(* Logix 5000 AddOnInstructionDefinition export AMCI_3601_AOP_Home_CCW; software revision 20.03 *)

ADD_ON_INSTRUCTION AMCI_3601_AOP_Home_CCW   (* revision 0.0, vendor AMCI, ExecuteEnableInFalse *)
// Revision note:
// 3/2020: Version 0 is the initial release
VAR_INPUT
   Axis_Status_Bits : INT; {required}
   Programmed_Speed : DINT; {required}
   Acceleration : INT; {required}
   Deceleration : INT; {required}
END_VAR
VAR_OUTPUT
   EN : BOOL; {access Read Only, visible}
   ER : BOOL; {access Read Only, visible}
END_VAR
VAR_IN_OUT
   AMCI_3601_output_data : AM:1769_3601:O:0; {required}
END_VAR
VAR
   Upper_Result_X_1000 : DINT;
   command_data_block : INT[10];
        [0]   // Command Bits MSW
        [1]   // Command Bits LSW
        [2]   // Upper Target Position
        [3]   // Lower Target Position
        [4]   // Upper Programmed Speed
        [5]   // Lower Programmed Speed
END_VAR

ROUTINE EnableInFalse   (* ladder *)
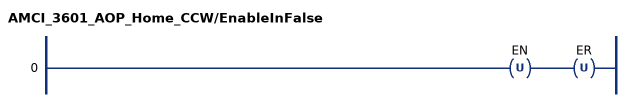
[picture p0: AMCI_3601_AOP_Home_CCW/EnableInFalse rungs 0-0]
   0: OTU(EN)OTU(ER);
END_ROUTINE

ROUTINE Logic   (* ladder *)
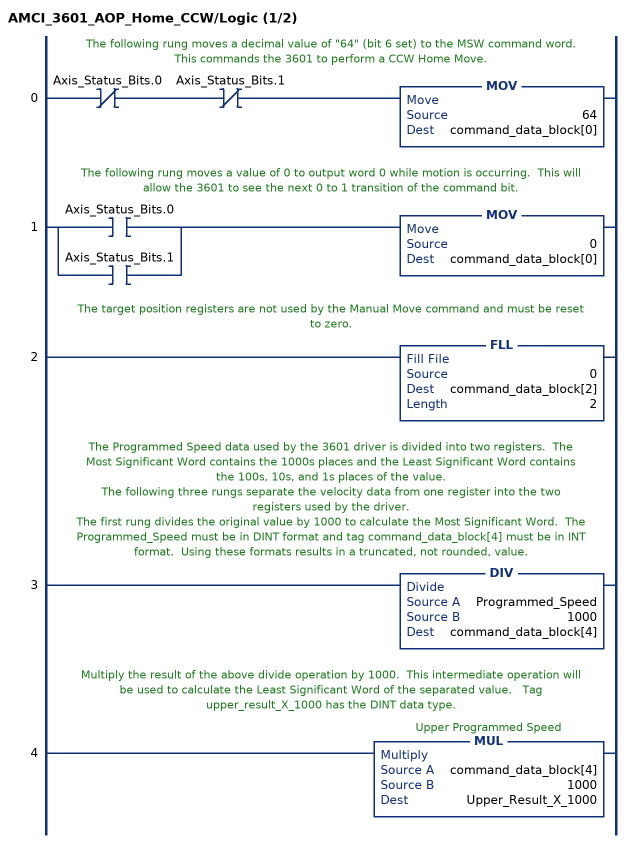
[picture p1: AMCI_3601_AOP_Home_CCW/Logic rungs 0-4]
   // The following rung moves a decimal value of "64" (bit 6 set) to the MSW command word.  This commands the 3601 to perform a CCW Home Move.
   0: XIO(Axis_Status_Bits.0)XIO(Axis_Status_Bits.1)MOV(64,command_data_block[0]);
   // The following rung moves a value of 0 to output word 0 while motion is occurring.  This will allow the 3601 to see the next 0 to 1 transition of the command bit.
   1: [XIC(Axis_Status_Bits.0) ,XIC(Axis_Status_Bits.1) ]MOV(0,command_data_block[0]);
   // The target position registers are not used by the Manual Move command and must be reset to zero.
   2: FLL(0,command_data_block[2],2);
   // The Programmed Speed data used by the 3601 driver is divided into two registers.  The Most Significant Word contains the 1000s places and the Least Significant Word contains the 100s, 10s, and 1s places of the value.
   // The following three rungs separate the velocity data from one register into the two registers used by the driver.
   // The first rung divides the original value by 1000 to calculate the Most Significant Word.  The Programmed_Speed must be in DINT format and tag command_data_block[4] must be in INT format.  Using these formats results in a truncated, not rounded, value.
   3: DIV(Programmed_Speed,1000,command_data_block[4]);
   // Multiply the result of the above divide operation by 1000.  This intermediate operation will be used to calculate the Least Significant Word of the separated value.   Tag upper_result_X_1000 has the DINT data type.
   4: MUL(command_data_block[4],1000,Upper_Result_X_1000);
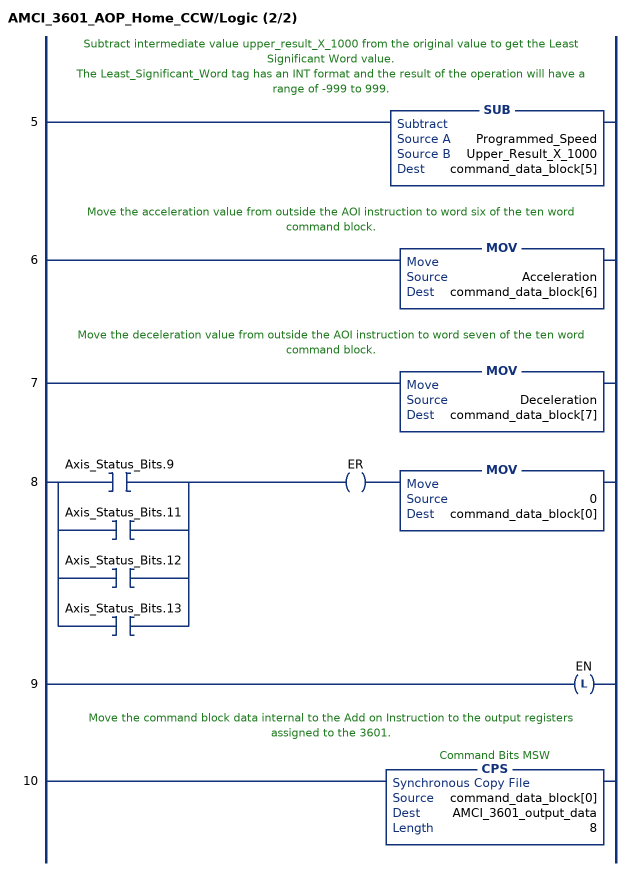
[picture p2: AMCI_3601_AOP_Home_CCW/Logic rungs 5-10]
   // Subtract intermediate value upper_result_X_1000 from the original value to get the Least Significant Word value.
   // The Least_Significant_Word tag has an INT format and the result of the operation will have a range of -999 to 999.
   5: SUB(Programmed_Speed,Upper_Result_X_1000,command_data_block[5]);
   // Move the acceleration value from outside the AOI instruction to word six of the ten word command block.
   6: MOV(Acceleration,command_data_block[6]);
   // Move the deceleration value from outside the AOI instruction to word seven of the ten word command block.
   7: MOV(Deceleration,command_data_block[7]);
   8: [XIC(Axis_Status_Bits.9) ,XIC(Axis_Status_Bits.11) ,XIC(Axis_Status_Bits.12) ,XIC(Axis_Status_Bits.13) ]OTE(ER)MOV(0,command_data_block[0]);
   9: OTL(EN);
   // Move the command block data internal to the Add on Instruction to the output registers assigned to the 3601.
   10: CPS(command_data_block[0],AMCI_3601_output_data,8);
END_ROUTINE
END_ADD_ON_INSTRUCTION
